(* Logix 5000 DataType export stSCTMi_Ejector; software revision 30.00 *)

TYPE stSCTMi_Ejector :
STRUCT
   siErrorByte : SINT;
   siWarningByte : SINT;
   siLeakageOfLastCycle : SINT;
   iSystemVacuum : INT;
   iEvacuationTimeT1 : INT;
   iLastFreeFlowVacuum : INT;
   iAirConsumptionOfLastCyc : INT;
   bAirSavingFunktion_H1 : BOOL;
   bPartPresent_H2 : BOOL;
END_STRUCT
END_TYPE
